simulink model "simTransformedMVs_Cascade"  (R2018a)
settings: Solver=ode15s  StartTime=0.0  StopTime=tsim  RelTol=1e-3
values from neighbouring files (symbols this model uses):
  dF = 1;0*F0    [TransformedMVs.m]
  dT = 1;0*T0    [TransformedMVs.m]
  dT1 = 0.15*T10    (= 3)    [TransformedMVs.m]
  dT2 = 0.1*T20    (= 5)    [TransformedMVs.m]
  F0 = 10    [TransformedMVs.m]
  Kc = 1/k.T*tau.T/(tauC.T+theta)    [TransformedMVs.m]    (also in Main.m = 1/k*tau/(tauC+theta); runTransf.m = 1/kM(i)*tau(i)/(tauCM(i)+theta(i)); runTransfOL.m = 1/kM(i)*tau(i)/(tauCM(i)+theta(i)))
  KI = 1/k.F/(tauC.F+theta)    [TransformedMVs.m]    (also in Main.m = Kp/tauIv; Main_OL.m = 1; runTransf.m = 1/kS(i)*1/tauCS(i); runTransfOL.m = 1/kS(i)*1/tauCS(i))
  T0 = 35    [hmeas.m]    (also in TransformedMVs.m; H2P_Turbine_driven.m = param(9); runTD.m = 318; H2P_Boiler_driven.m = param(9))
  T10 = 20    [TransformedMVs.m]
  T20 = 50    [TransformedMVs.m]
  tauI = min(tau.T,4*(tauC.T+theta))    [TransformedMVs.m]    (also in Main.m = min(tau,4*(tauC+theta)); runTransf.m = min(tau(i), 4*(tauCM(i)+theta(i))); runTransfOL.m = min(tau(i), 4*(tauCM(i)+theta(i))))
  tstep_F = 200    [TransformedMVs.m]
  tstep_T = 150    [TransformedMVs.m]
  v1_0 = F10+F20    (= 10)    [TransformedMVs.m]
  v2_0 = tau0/m*(F10*T10+F20*T20)+(1-tau0/taur0)*T0    (= 35)    [TransformedMVs.m]
undefined symbols (not defined in the file or in its folder): Kc_F, shower, tstep_d, u1_0, u2_0, utmeasured
libraries: simulink x4

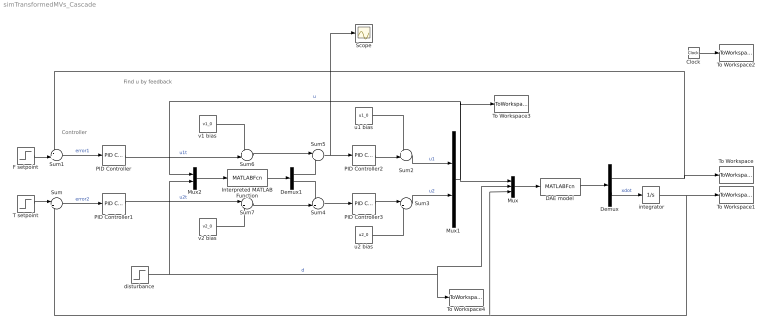
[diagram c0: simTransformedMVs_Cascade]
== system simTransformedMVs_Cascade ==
  note: Controller
  note: Find u by feedback
  " integrator" : Integrator  InitialCondition=T0
  Clock : Clock
  DAE model : MATLABFcn  MATLABFcn=shower(u(1:2), u(3:4),u(5))  OutputDimensions=2
  Demux : Demux  Outputs=2
  Demux1 : Demux  Outputs=2
  F setpoint : Step  Time=tstep_F  Before=F0  After=F0+dF  SampleTime=0
  Interpreted MATLAB Function : MATLABFcn  MATLABFcn=utmeasured(u(1:2),u(3:4))  OutputDimensions=2
  Mux : Mux  Inputs=3
  Mux1 : Mux  Inputs=2
  Mux2 : Mux  Inputs=2
  PID Controller : simulink/Continuous/PID Controller  Controller=I  TimeDomain=Continuous-time  SampleTime=-1  IntegratorMethod=Forward Euler  FilterMethod=Forward Euler  Form=Ideal  UseFilter=on  ControllerParametersSource=internal  P=Kc_F  I=KI  D=0  N=100  InitialConditionSource=internal  InitialConditionForIntegrator=0  InitialConditionForFilter=0  ExternalReset=none  LimitOutput=off  UpperSaturationLimit=inf  LowerSaturationLimit=-inf  LinearizeAsGain=on  AntiWindupMode=none  Kb=1  TrackingMode=off  Kt=1  PParamMin=[]  PParamMax=[]  IParamMin=[]  IParamMax=[]  DParamMin=[]  DParamMax=[]  NParamMin=[]  NParamMax=[]  KbParamMin=[]  KbParamMax=[]  KtParamMin=[]  KtParamMax=[]  POutMin=[]  POutMax=[]  IOutMin=[]  IOutMax=[]  DOutMin=[]  DOutMax=[]  NOutMin=[]  NOutMax=[]  KbOutMin=[]  KbOutMax=[]  KtOutMin=[]  KtOutMax=[]  IntegratorOutMin=[]  IntegratorOutMax=[]  FilterOutMin=[]  FilterOutMax=[]  SumOutMin=[]  SumOutMax=[]  SumI1OutMin=[]  SumI1OutMax=[]  SumI2OutMin=[]  SumI2OutMax=[]  SumI3OutMin=[]  SumI3OutMax=[]  SumDOutMin=[]  SumDOutMax=[]  SaturationOutMin=[]  SaturationOutMax=[]  IntegratorContinuousStateAttributes=''  IntegratorStateMustResolveToSignalObject=off  IntegratorRTWStateStorageClass=Auto  FilterContinuousStateAttributes=''  FilterStateMustResolveToSignalObject=off  FilterRTWStateStorageClass=Auto  DifferentiatorICPrevScaledInput=0  DifferentiatorOutMin=[]  DifferentiatorOutMax=[]  FilterDiffOutCoefMin=[]  FilterDiffOutCoefMax=[]  SumDenOutMin=[]  SumDenOutMax=[]  SumNumOutMin=[]  SumNumOutMax=[]  ReciprocalOutMin=[]  ReciprocalOutMax=[]  DivideOutMin=[]  DivideOutMax=[]  TunerSelectOption=Transfer Function Based (PID Tuner App)
  PID Controller1 : simulink/Continuous/PID Controller  Controller=PI  TimeDomain=Continuous-time  SampleTime=-1  IntegratorMethod=Forward Euler  FilterMethod=Forward Euler  Form=Ideal  UseFilter=on  ControllerParametersSource=internal  P=Kc  I=1/tauI  D=0  N=100  InitialConditionSource=internal  InitialConditionForIntegrator=0  InitialConditionForFilter=0  ExternalReset=none  LimitOutput=off  UpperSaturationLimit=inf  LowerSaturationLimit=-inf  LinearizeAsGain=on  AntiWindupMode=none  Kb=1  TrackingMode=off  Kt=1  PParamMin=[]  PParamMax=[]  IParamMin=[]  IParamMax=[]  DParamMin=[]  DParamMax=[]  NParamMin=[]  NParamMax=[]  KbParamMin=[]  KbParamMax=[]  KtParamMin=[]  KtParamMax=[]  POutMin=[]  POutMax=[]  IOutMin=[]  IOutMax=[]  DOutMin=[]  DOutMax=[]  NOutMin=[]  NOutMax=[]  KbOutMin=[]  KbOutMax=[]  KtOutMin=[]  KtOutMax=[]  IntegratorOutMin=[]  IntegratorOutMax=[]  FilterOutMin=[]  FilterOutMax=[]  SumOutMin=[]  SumOutMax=[]  SumI1OutMin=[]  SumI1OutMax=[]  SumI2OutMin=[]  SumI2OutMax=[]  SumI3OutMin=[]  SumI3OutMax=[]  SumDOutMin=[]  SumDOutMax=[]  SaturationOutMin=[]  SaturationOutMax=[]  IntegratorContinuousStateAttributes=''  IntegratorStateMustResolveToSignalObject=off  IntegratorRTWStateStorageClass=Auto  FilterContinuousStateAttributes=''  FilterStateMustResolveToSignalObject=off  FilterRTWStateStorageClass=Auto  DifferentiatorICPrevScaledInput=0  DifferentiatorOutMin=[]  DifferentiatorOutMax=[]  FilterDiffOutCoefMin=[]  FilterDiffOutCoefMax=[]  SumDenOutMin=[]  SumDenOutMax=[]  SumNumOutMin=[]  SumNumOutMax=[]  ReciprocalOutMin=[]  ReciprocalOutMax=[]  DivideOutMin=[]  DivideOutMax=[]  TunerSelectOption=Transfer Function Based (PID Tuner App)
  PID Controller2 : simulink/Continuous/PID Controller  Controller=PI  TimeDomain=Continuous-time  SampleTime=-1  IntegratorMethod=Forward Euler  FilterMethod=Forward Euler  Form=Ideal  UseFilter=on  ControllerParametersSource=internal  P=1  I=1/000.1  D=0  N=100  InitialConditionSource=internal  InitialConditionForIntegrator=0  InitialConditionForFilter=0  ExternalReset=none  LimitOutput=off  UpperSaturationLimit=inf  LowerSaturationLimit=-inf  LinearizeAsGain=on  AntiWindupMode=none  Kb=1  TrackingMode=off  Kt=1  PParamMin=[]  PParamMax=[]  IParamMin=[]  IParamMax=[]  DParamMin=[]  DParamMax=[]  NParamMin=[]  NParamMax=[]  KbParamMin=[]  KbParamMax=[]  KtParamMin=[]  KtParamMax=[]  POutMin=[]  POutMax=[]  IOutMin=[]  IOutMax=[]  DOutMin=[]  DOutMax=[]  NOutMin=[]  NOutMax=[]  KbOutMin=[]  KbOutMax=[]  KtOutMin=[]  KtOutMax=[]  IntegratorOutMin=[]  IntegratorOutMax=[]  FilterOutMin=[]  FilterOutMax=[]  SumOutMin=[]  SumOutMax=[]  SumI1OutMin=[]  SumI1OutMax=[]  SumI2OutMin=[]  SumI2OutMax=[]  SumI3OutMin=[]  SumI3OutMax=[]  SumDOutMin=[]  SumDOutMax=[]  SaturationOutMin=[]  SaturationOutMax=[]  IntegratorContinuousStateAttributes=''  IntegratorStateMustResolveToSignalObject=off  IntegratorRTWStateStorageClass=Auto  FilterContinuousStateAttributes=''  FilterStateMustResolveToSignalObject=off  FilterRTWStateStorageClass=Auto  DifferentiatorICPrevScaledInput=0  DifferentiatorOutMin=[]  DifferentiatorOutMax=[]  FilterDiffOutCoefMin=[]  FilterDiffOutCoefMax=[]  SumDenOutMin=[]  SumDenOutMax=[]  SumNumOutMin=[]  SumNumOutMax=[]  ReciprocalOutMin=[]  ReciprocalOutMax=[]  DivideOutMin=[]  DivideOutMax=[]  TunerSelectOption=Transfer Function Based (PID Tuner App)
  PID Controller3 : simulink/Continuous/PID Controller  Controller=PI  TimeDomain=Continuous-time  SampleTime=-1  IntegratorMethod=Forward Euler  FilterMethod=Forward Euler  Form=Ideal  UseFilter=on  ControllerParametersSource=internal  P=1  I=1/000.1  D=0  N=100  InitialConditionSource=internal  InitialConditionForIntegrator=0  InitialConditionForFilter=0  ExternalReset=none  LimitOutput=off  UpperSaturationLimit=inf  LowerSaturationLimit=-inf  LinearizeAsGain=on  AntiWindupMode=none  Kb=1  TrackingMode=off  Kt=1  PParamMin=[]  PParamMax=[]  IParamMin=[]  IParamMax=[]  DParamMin=[]  DParamMax=[]  NParamMin=[]  NParamMax=[]  KbParamMin=[]  KbParamMax=[]  KtParamMin=[]  KtParamMax=[]  POutMin=[]  POutMax=[]  IOutMin=[]  IOutMax=[]  DOutMin=[]  DOutMax=[]  NOutMin=[]  NOutMax=[]  KbOutMin=[]  KbOutMax=[]  KtOutMin=[]  KtOutMax=[]  IntegratorOutMin=[]  IntegratorOutMax=[]  FilterOutMin=[]  FilterOutMax=[]  SumOutMin=[]  SumOutMax=[]  SumI1OutMin=[]  SumI1OutMax=[]  SumI2OutMin=[]  SumI2OutMax=[]  SumI3OutMin=[]  SumI3OutMax=[]  SumDOutMin=[]  SumDOutMax=[]  SaturationOutMin=[]  SaturationOutMax=[]  IntegratorContinuousStateAttributes=''  IntegratorStateMustResolveToSignalObject=off  IntegratorRTWStateStorageClass=Auto  FilterContinuousStateAttributes=''  FilterStateMustResolveToSignalObject=off  FilterRTWStateStorageClass=Auto  DifferentiatorICPrevScaledInput=0  DifferentiatorOutMin=[]  DifferentiatorOutMax=[]  FilterDiffOutCoefMin=[]  FilterDiffOutCoefMax=[]  SumDenOutMin=[]  SumDenOutMax=[]  SumNumOutMin=[]  SumNumOutMax=[]  ReciprocalOutMin=[]  ReciprocalOutMax=[]  DivideOutMin=[]  DivideOutMax=[]  TunerSelectOption=Transfer Function Based (PID Tuner App)
  Scope : Scope
  Sum : Sum  Inputs=|+-
  Sum1 : Sum  Inputs=-+|
  Sum2 : Sum  Inputs=++|
  Sum3 : Sum  Inputs=|++
  Sum4 : Sum  Inputs=-+|
  Sum5 : Sum  Inputs=|+-
  Sum6 : Sum  Inputs=++|
  Sum7 : Sum  Inputs=|++
  T setpoint : Step  Time=tstep_T  Before=T0  After=T0+dT  SampleTime=0
  To Workspace : ToWorkspace  VariableName=F  SampleTime=-1
  To Workspace1 : ToWorkspace  VariableName=T  SampleTime=-1
  To Workspace2 : ToWorkspace  VariableName=time  SampleTime=-1
  To Workspace3 : ToWorkspace  VariableName=u  SampleTime=-1
  To Workspace4 : ToWorkspace  VariableName=d  SampleTime=-1
  disturbance : Step  Time=tstep_d  Before=[T10;T20]  After=[T10+dT1; T20+dT2]  SampleTime=0
  u1 bias : Constant  Value=u1_0
  u2 bias : Constant  Value=u2_0
  v1 bias : Constant  Value=v1_0
  v2 bias : Constant  Value=v2_0
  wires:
  DAE model/1 -> Demux/1
  Demux/1 -> To Workspace/1, Sum1/1  "T"
  " integrator"/1 -> To Workspace1/1, Mux/3, Sum/2  "T"
  Mux/1 -> DAE model/1
  Clock/1 -> To Workspace2/1
  disturbance/1 -> Mux2/2, To Workspace4/1, Mux/2  "d"
  Sum/1 -> PID Controller1/1  "error2"
  T setpoint/1 -> Sum/1
  Sum1/1 -> PID Controller/1  "error1"
  F setpoint/1 -> Sum1/2
  Mux1/1 -> Mux2/1, To Workspace3/1, Mux/1  "u"
  PID Controller/1 -> Sum6/2  "u1t"
  PID Controller1/1 -> Sum7/1  "u2t"
  u2 bias/1 -> Sum3/2
  Demux/2 -> " integrator"/1  "xdot"
  PID Controller2/1 -> Sum2/2
  PID Controller3/1 -> Sum3/1
  u1 bias/1 -> Sum2/1
  Sum2/1 -> Mux1/1  "u1"
  Sum3/1 -> Mux1/2  "u2"
  Sum4/1 -> PID Controller3/1
  Sum5/1 -> Scope/1, PID Controller2/1
  Mux2/1 -> Interpreted MATLAB Function/1
  Interpreted MATLAB Function/1 -> Demux1/1
  Demux1/1 -> Sum5/2
  Demux1/2 -> Sum4/1
  v1 bias/1 -> Sum6/1
  v2 bias/1 -> Sum7/2
  Sum6/1 -> Sum5/1
  Sum7/1 -> Sum4/2
